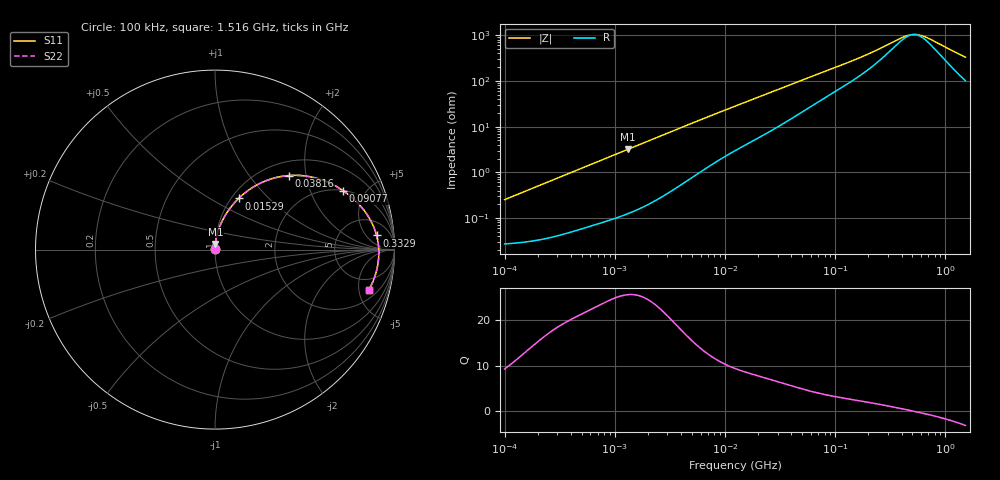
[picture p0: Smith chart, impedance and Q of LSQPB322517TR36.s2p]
! LSQPB322517TR36  S-PARAMETER MODEL  ( General Type )
! Model Generated by TAIYO YUDEN Corporation (http://www.ty-top.com)
! Version 1.0
! TAIYO YUDEN Control No. 100901NG22SB-FKC
! Copyright(c) 2010 TAIYO YUDEN CO.,LTD. All Rights Reserved.
! Product Description (link to TY-COMPAS)
! https://ds.yuden.co.jp/TYCOMPAS/or/detail?pn=LSQPB322517TR36M&u=M
! Products Name : Inductors
! Characteristics :
!  Inductance : 0.36 uH , SRF(min) : 350 MHz , DC Resistance(max) : 0.0325 Ohm
!  Rated Current : Saturation :4300 mA , Temp Rise : 2750 mA (40 degC)
!  Case Size : 3.2 x 2.5 / 0.126 x 0.098 [mm/inch] , Thickness : 1.7 / 0.068 [mm/inch]
!  (Conditions: Temperature = 25 degC , DC Bias Current/Voltage = 0A / 0V)
! External Node Assignments :
!  1  o---GGG---o  2
! GND o---------o GND
! Frequency Range : 0.1MHz  -  1516.370183MHz  [ 402 STEP ]
# MHz S RI R 50
! Freq[MHz].  S11 Real  S11 Imag  S21 Real  S21 Imag  S12 Real  S12 Imag  S22 Real  S22 Imag
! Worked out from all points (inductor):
!   401 points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, 100 kHz to 1.516 GHz, reference 50 ohm
!   read as one part in series: L = 399 nH near 104.9 kHz
!   highest Q = 25.6 at 1.313 MHz (marker M1), where L = 386 nH
!   self-resonance near 514 MHz
!   S11 on the Smith chart (normalised r, x): 100 kHz: 1.00, +0.01; 15.29 MHz: 1.08, +0.68; 38.16 MHz: 1.28, +1.60; 90.77 MHz: 2.02, +3.47; 332.9 MHz: 11, +10; 1.516 GHz: 3.03, -6.34
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0.1  0.000277 0.00251  0.9997 -0.00251  0.9997 -0.00251  0.000277 0.00251
0.501516  0.000732 0.0124  0.9993 -0.0124  0.9993 -0.0124  0.000732 0.0124
1.313304  0.00225 0.0317  0.9977 -0.0317  0.9977 -0.0317  0.00225 0.0317
2.515184  0.00627 0.06  0.9937 -0.06  0.9937 -0.06  0.00627 0.06
6.429812  0.0329 0.1445  0.9671 -0.1445  0.9671 -0.1445  0.0329 0.1445
12.61405  0.0988 0.2494  0.9012 -0.2494  0.9012 -0.2494  0.0988 0.2494
15.29223  0.1318 0.285  0.8682 -0.285  0.8682 -0.285  0.1318 0.285
23.58343  0.2395 0.3634  0.7605 -0.3634  0.7605 -0.3634  0.2395 0.3634
38.16342  0.4125 0.4128  0.5875 -0.4128  0.5875 -0.4128  0.4125 0.4128
48.54756  0.5075 0.4096  0.4925 -0.4096  0.4925 -0.4096  0.5075 0.4096
61.75718  0.5967 0.3879  0.4033 -0.3879  0.4033 -0.3879  0.5967 0.3879
90.76527  0.7147 0.3278  0.2853 -0.3278  0.2853 -0.3278  0.7147 0.3278
124.1069  0.7862 0.2686  0.2138 -0.2686  0.2138 -0.2686  0.7862 0.2686
173.8297  0.8421 0.2025  0.1579 -0.2025  0.1579 -0.2025  0.8421 0.2025
309.7222  0.8967 0.0919  0.1033 -0.0919  0.1033 -0.0919  0.8967 0.0919
332.9112  0.9005 0.0786  0.0995 -0.0786  0.0995 -0.0786  0.9005 0.0786
455.2024  0.9108 0.0219  0.0892 -0.0219  0.0892 -0.0219  0.9108 0.0219
513.4104  0.9124 0.000216  0.0876 -0.000216  0.0876 -0.000216  0.9124 0.000216
579.0615  0.9128 -0.0217  0.0872 0.0217  0.0872 0.0217  0.9128 -0.0217
702.006  0.9107 -0.0576  0.0893 0.0576  0.0893 0.0576  0.9107 -0.0576
1192.024  0.8841 -0.1675  0.1159 0.1675  0.1159 0.1675  0.8841 -0.1675
1516.37  0.8571 -0.2249  0.1429 0.2249  0.1429 0.2249  0.8571 -0.2249
